(* Logix 5000 AddOnInstructionDefinition export AMCI_SMD23E2_Registration_Move_CCW; software revision 20.03 *)

ADD_ON_INSTRUCTION AMCI_SMD23E2_Registration_Move_CCW   (* revision 1.0, vendor AMCI *)
VAR_INPUT
   Type_0_for_standard_1_for_indexed : BOOL;
   Stopping_Distance : DINT; {required}
   Programmed_Speed : DINT; {required}
   Acceleration : INT; {required}
   Deceleration : INT; {required}
   Minimum_Registration_Move_Distance : DINT; {required}
END_VAR
VAR_OUTPUT
   Registration_Move_CCW_Occurring : BOOL; {access Read Only, visible}
END_VAR
VAR_IN_OUT
   AMCI_SMD23E2_output_data : _000A:SMD23E2_788832CB:O:0; {required}
END_VAR
VAR
   Upper_Result_X_1000 : DINT;
   command_data_block : INT[10];
        [0]   // Command Bits MSW
        [1]   // Command Bits LSW
        [2]   // Upper Target Position
        [3]   // Lower Target Position
        [4]   // Upper Programmed Speed
        [5]   // Lower Programmed Speed
END_VAR

ROUTINE Logic   (* ladder *)
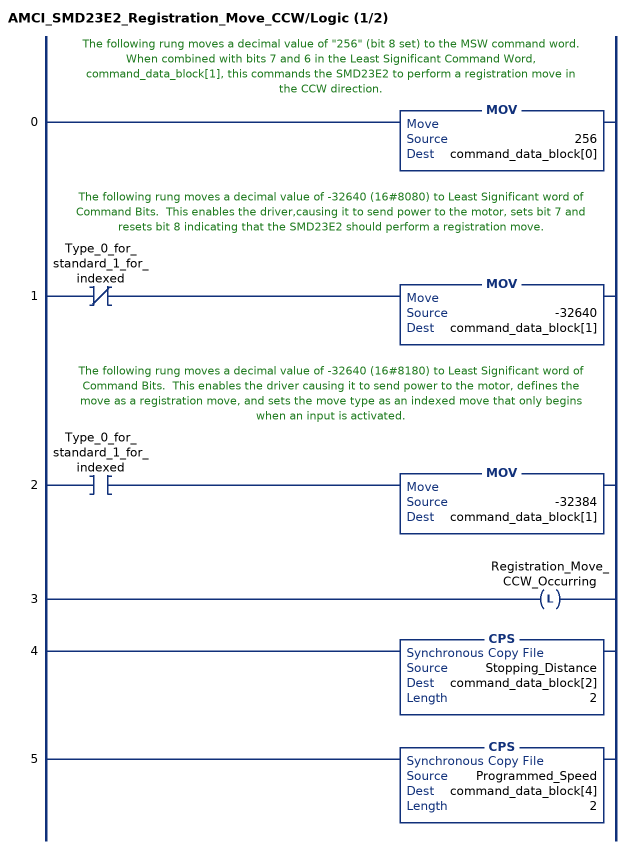
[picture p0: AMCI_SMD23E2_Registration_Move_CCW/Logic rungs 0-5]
   // The following rung moves a decimal value of "256" (bit 8 set) to the MSW command word.  When combined with bits 7 and 6 in the Least Significant Command Word, command_data_block[1], this commands the SMD23E2 to perform a registration move in the CCW direction.
   0: MOV(256,command_data_block[0]);
   // The following rung moves a decimal value of -32640 (16#8080) to Least Significant word of Command Bits.  This enables the driver,causing it to send power to the motor, sets bit 7 and resets bit 8 indicating that the SMD23E2 should perform a registration move.
   1: XIO(Type_0_for_standard_1_for_indexed)MOV(-32640,command_data_block[1]);
   // The following rung moves a decimal value of -32640 (16#8180) to Least Significant word of Command Bits.  This enables the driver causing it to send power to the motor, defines the move as a registration move, and sets the move type as an indexed move that only begins when an input is activated.
   2: XIC(Type_0_for_standard_1_for_indexed)MOV(-32384,command_data_block[1]);
   3: OTL(Registration_Move_CCW_Occurring);
   4: CPS(Stopping_Distance,command_data_block[2],2);
   5: CPS(Programmed_Speed,command_data_block[4],2);
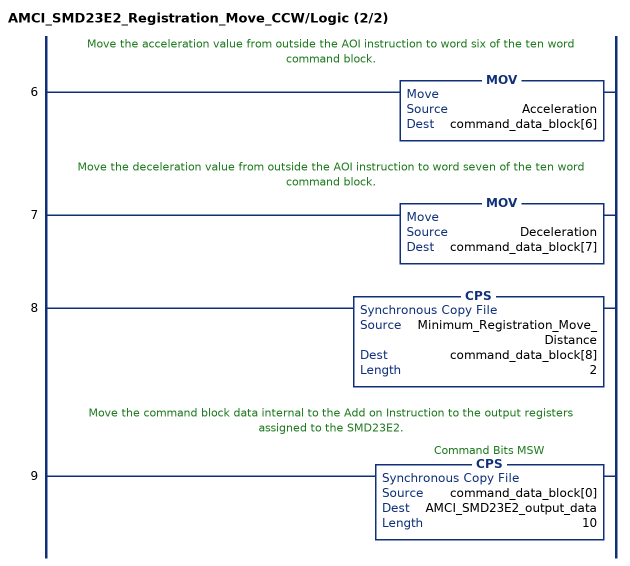
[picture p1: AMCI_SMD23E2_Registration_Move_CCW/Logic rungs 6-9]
   // Move the acceleration value from outside the AOI instruction to word six of the ten word command block.
   6: MOV(Acceleration,command_data_block[6]);
   // Move the deceleration value from outside the AOI instruction to word seven of the ten word command block.
   7: MOV(Deceleration,command_data_block[7]);
   8: CPS(Minimum_Registration_Move_Distance,command_data_block[8],2);
   // Move the command block data internal to the Add on Instruction to the output registers assigned to the SMD23E2.
   9: CPS(command_data_block[0],AMCI_SMD23E2_output_data,10);
END_ROUTINE
END_ADD_ON_INSTRUCTION
